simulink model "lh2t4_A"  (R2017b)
settings: Solver=ode45  StartTime=0.0  StopTime=10  RelTol=1e-3  EnableMultiTasking=on
libraries: mat24129_lib x1

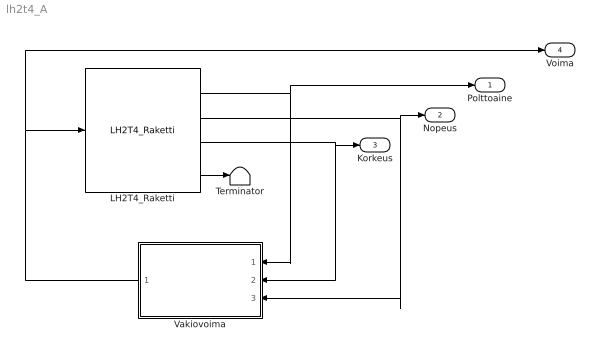
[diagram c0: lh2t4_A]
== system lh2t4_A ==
  LH2T4_Raketti : mat24129_lib/LH2T4_Raketti
  Terminator : Terminator
  Vakiovoima : Subsystem
  Polttoaine : Outport
  Nopeus : Outport  Port=2
  Korkeus : Outport  Port=3
  Voima : Outport  Port=4
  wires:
  LH2T4_Raketti/1 -> Polttoaine/1, Vakiovoima/1(Polttoaine)
  LH2T4_Raketti/2 -> Nopeus/1, Vakiovoima/3(Nopeus)
  LH2T4_Raketti/3 -> Korkeus/1, Vakiovoima/2(Korkeus)
  Vakiovoima/1(Voima) -> Voima/1, LH2T4_Raketti/1
  LH2T4_Raketti/4 -> Terminator/1

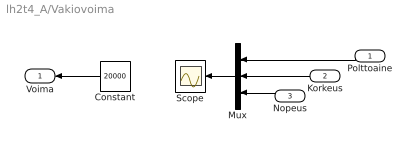
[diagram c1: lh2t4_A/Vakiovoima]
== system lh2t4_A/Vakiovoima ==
  Polttoaine : Inport
  Korkeus : Inport  Port=2
  Nopeus : Inport  Port=3
  Constant : Constant  Value=20000
  Mux : Mux  Inputs=3
  Scope : Scope
  Voima : Outport
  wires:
  Mux/1 -> Scope/1
  Korkeus/1 -> Mux/2
  Nopeus/1 -> Mux/3
  Constant/1 -> Voima/1
  Polttoaine/1 -> Mux/1
